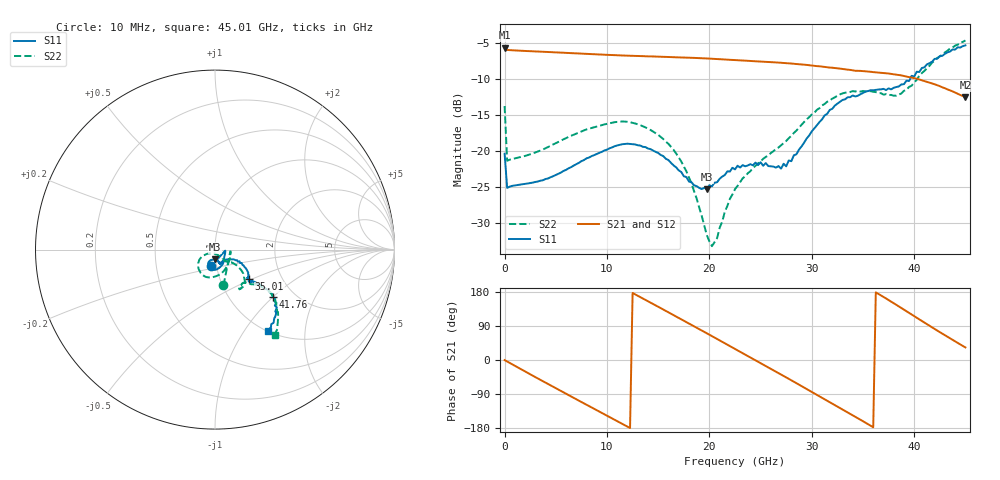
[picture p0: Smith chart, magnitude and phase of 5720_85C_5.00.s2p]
! Device:  ADRF5720
! Description: 0.5dB LSB GaAs MMIC 6-bit Digital Attenuator
! Frequency:  0.000009 -  40 GHz
! Ports:
!	RF1	= Port 1
!	RF2	= Port 2
! Vdd:  3.3 Volt
! Vss:  -3.3 Volt
! Control:  0/3.3 Volt
! State:  5.00 dB attenuation
! Data:  The device was measured using G-S-G Probes on a matrix board.
!  Data was collected using an calibrated 4 port network analyzer.
!  The reference plane for this measurement is at the launchers.
! Note:  Analog Devices supplies this data as a sample of measured data
!  for this product.  Your particular data for this product may vary.
!  Data was taken at 85 degrees C.
!  Analog Devices reserves the right to change this data at anytime.
# GHZ S DB R 45.0
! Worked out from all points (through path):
!   181 points, 10 MHz to 45.01 GHz, reference 45 ohm
!   highest |S21| = -5.70 dB at 10 MHz (marker M1); lowest = -12.6 dB at 45.01 GHz (marker M2)
!   group delay of S21, straight-line fit = 42 ps
!   lowest |S11| = -25.3 dB at 19.76 GHz (marker M3), VSWR 1.12, Z = 44.9 - j4.91 ohm
!   |S11| at or under -10 dB: start of sweep to 39.61 GHz
!   |S22| runs from -33.1 to -4.7 dB; largest |S21 - S12| = 0.0026
!   S11 on the Smith chart (normalised r, x): 10 MHz: 0.94, -0.18; 35.01 GHz: 1.37, -0.49; 41.76 GHz: 1.57, -1.00; 45.01 GHz: 1.01, -1.29
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0.01  -20.36 -102.9  -5.70 -0.3  -5.68 -0.3  -13.76 -76.7
0.26  -25.08 -8.4  -6.00 -4.0  -5.99 -4.0  -21.33 -6.5
2.01  -24.52 -16.2  -6.14 -30.4  -6.12 -30.3  -20.66 -20.9
4.26  -23.77 -36.6  -6.29 -63.5  -6.27 -63.4  -19.43 -46.7
7.76  -21.23 -57.7  -6.52 -114.5  -6.51 -114.4  -17.13 -76.8
11.51  -19.04 -87.0  -6.77 -168.7  -6.75 -168.6  -15.90 -107.9
13.26  -19.22 -100.6  -6.85 166.0  -6.84 166.1  -16.40 -122.4
15.26  -20.53 -113.0  -6.94 136.8  -6.92 137.0  -18.04 -138.7
17.76  -23.58 -112.8  -7.07 100.1  -7.05 100.3  -22.78 -152.7
19.76  -25.26 -88.5  -7.18 70.4  -7.17 70.6  -31.62 -130.0
20.26  -24.87 -83.7  -7.22 63.0  -7.20 63.2  -33.14 -104.5
20.76  -24.30 -79.8  -7.25 55.6  -7.24 55.8  -32.04 -79.3
22.76  -22.01 -71.4  -7.41 25.8  -7.39 26.0  -24.80 -50.6
25.01  -21.54 -68.7  -7.60 -8.0  -7.58 -7.7  -21.40 -48.7
27.51  -22.10 -46.1  -7.83 -45.9  -7.81 -45.6  -18.59 -37.2
30.26  -16.85 -27.7  -8.20 -88.3  -8.18 -88.0  -14.69 -38.0
32.26  -13.70 -31.9  -8.50 -119.0  -8.48 -118.8  -12.56 -45.6
35.01  -11.95 -40.9  -8.93 -161.6  -8.91 -161.2  -11.67 -57.2
37.76  -11.46 -40.4  -9.32 153.9  -9.30 154.3  -12.22 -52.4
39.76  -9.58 -38.2  -9.81 120.1  -9.79 120.5  -10.95 -43.0
41.76  -7.62 -39.2  -10.65 86.3  -10.63 86.7  -7.76 -38.5
45.01  -5.37 -56.8  -12.55 33.2  -12.52 33.5  -4.69 -54.9
